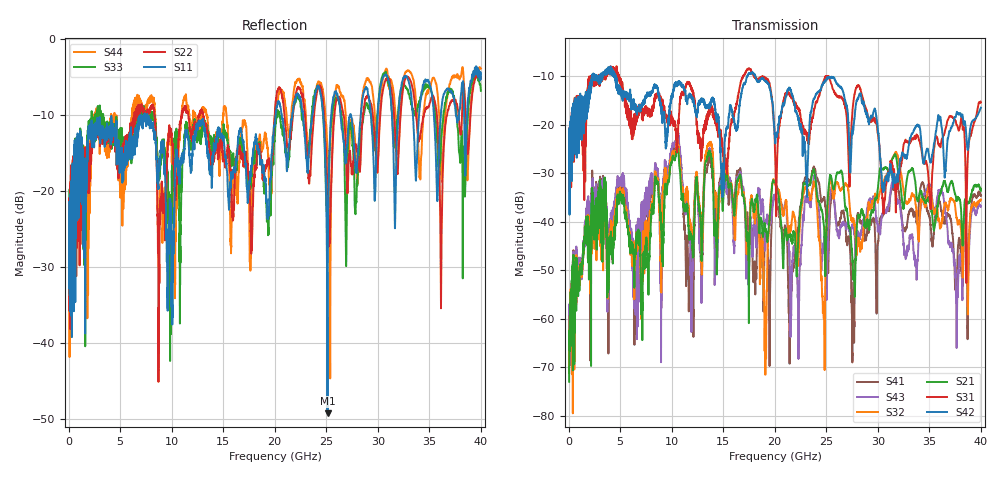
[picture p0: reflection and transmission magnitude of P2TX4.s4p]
!Agilent Technologies,N5245A,MY49151084,A.09.20.08
!Agilent N5245A: A.09.20.08
!Date: Thursday, March 01, 2012 11:54:21
!Correction: S11(Full 4 Port(1,2,3,4))
!S12(Full 4 Port(1,2,3,4))
!S13(Full 4 Port(1,2,3,4))
!S14(Full 4 Port(1,2,3,4))
!S21(Full 4 Port(1,2,3,4))
!S22(Full 4 Port(1,2,3,4))
!S23(Full 4 Port(1,2,3,4))
!S24(Full 4 Port(1,2,3,4))
!S31(Full 4 Port(1,2,3,4))
!S32(Full 4 Port(1,2,3,4))
!S33(Full 4 Port(1,2,3,4))
!S34(Full 4 Port(1,2,3,4))
!S41(Full 4 Port(1,2,3,4))
!S42(Full 4 Port(1,2,3,4))
!S43(Full 4 Port(1,2,3,4))
!S44(Full 4 Port(1,2,3,4))
!S4P File: Measurements: <S11,S12,S13,S14>,
!<S21,S22,S23,S24>,
!<S31,S32,S33,S34>,
!<S41,S42,S43,S44>:
# Hz S  dB  R 50
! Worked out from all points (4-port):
!   3996 points, 50 MHz to 40 GHz, reference 50 ohm
!   strongest paths, dB at 50 MHz, 10.04 GHz, 20.03 GHz, 30.02 GHz, 40 GHz:
!     S42: -23.6, -13.8, -22.9, -21.4, -16.5
!     S31: -24.9, -19.6, -24.8, -22.1, -15.4
!     S21: -73.0, -27.4, -31.7, -33.0, -33.6
!     S32: -69.6, -26.8, -32.2, -35.7, -35.4
!     S43: -64.5, -24.8, -34.7, -41.1, -36.9
!     S41: -71.2, -25.7, -34.8, -44.4, -34.7
!   lowest |S11| = -49.3 dB at 25.12 GHz (marker M1), VSWR 1.01, Z = 50.1 - j0.328 ohm
!   |S11| at or under -10 dB: start of sweep to 6.94 GHz; 7.633 GHz to 20.08 GHz (12.45 GHz wide, 89.8 % of centre); 20.69 GHz to 21.7 GHz (1.012 GHz wide, 4.77 % of centre)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
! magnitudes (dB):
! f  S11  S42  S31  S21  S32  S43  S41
! 50 MHz  -25.0  -23.6  -24.9  -73.0  -69.6  -64.5  -71.2
! 10.53 GHz  -15.3  -11.6  -25.7  -25.0  -23.4  -21.6  -23.1
! 11.92 GHz  -16.9  -14.3  -12.3  -43.5  -41.9  -62.7  -45.2
! 19.09 GHz  -18.4  -11.0  -10.4  -41.6  -71.6  -40.5  -43.3
! 19.87 GHz  -12.8  -18.2  -18.0  -31.4  -31.2  -35.3  -35.0
! 25.12 GHz  -49.3  -10.2  -10.0  -36.0  -38.0  -46.9  -43.9
! 40 GHz  -5.2  -16.5  -15.4  -33.6  -35.4  -36.9  -34.7
